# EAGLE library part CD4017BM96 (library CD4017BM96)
CMOS Decade Counter with 10 Decoded Outputs 16-SOIC -55 to 125
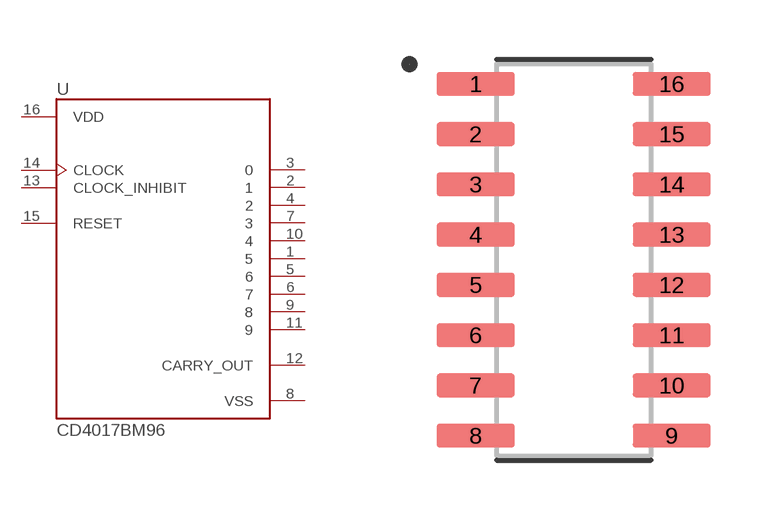
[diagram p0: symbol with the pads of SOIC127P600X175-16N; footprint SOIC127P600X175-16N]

Designator prefix U

## CD4017BM96 (MANUFACTURER: Texas Instruments; MAXIMUM_PACKAGE_HEIGHT: 1.75mm; PARTREV: Feb 2004; STANDARD: IPC-7351B)  [SOIC127P600X175-16N]
1  5  out
2  1  out
3  0  out
4  2  out
5  6  out
6  7  out
7  3  out
8  VSS  pwr
9  8  out
10  4  out
11  9  out
12  CARRY_OUT  out
13  CLOCK_INHIBIT  in
14  CLOCK  in
15  RESET  in
16  VDD  pwr

## Footprint SOIC127P600X175-16N (pad centres in mm)
smd 1.97 x 0.6: 1 -2.475,4.445; 2 -2.475,3.175; 3 -2.475,1.905; 4 -2.475,0.635; 5 -2.475,-0.635; 6 -2.475,-1.905; 7 -2.475,-3.175; 8 -2.475,-4.445; 9 2.475,-4.445; 10 2.475,-3.175; 11 2.475,-1.905; 12 2.475,-0.635; 13 2.475,0.635; 14 2.475,1.905; 15 2.475,3.175; 16 2.475,4.445

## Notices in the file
This work is licensed under a Creative Commons Attribution-ShareAlike 4.0 International License (CC BY-SA) with Design Exception 1.0
